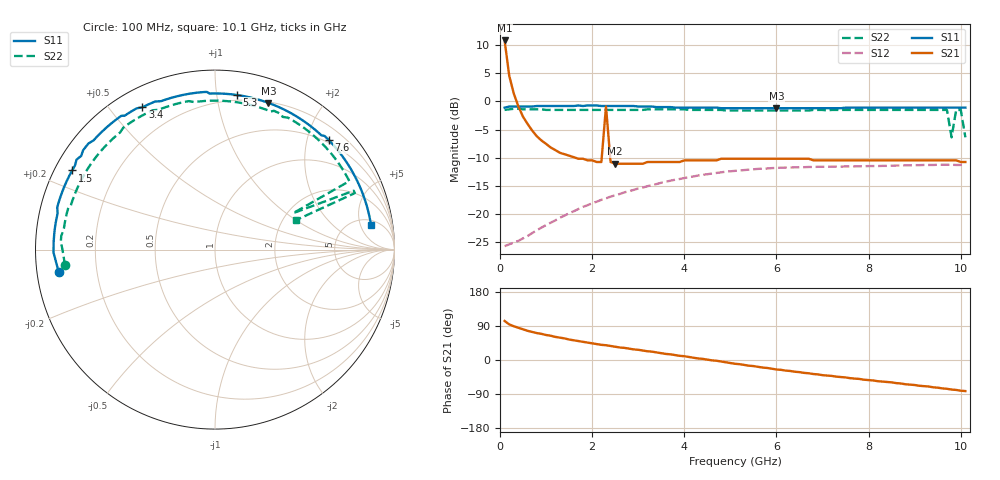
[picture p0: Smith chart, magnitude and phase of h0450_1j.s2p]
!HBFP-0450
!S and NOISE PARAMETERS at Vce=1V  Ic=100mA.  LAST UPDATED  09-04-98
# GHZ S MA R  50
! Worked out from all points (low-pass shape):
!   101 points, 100 MHz to 10.1 GHz, reference 50 ohm
!   highest |S21| = 10.81 dB at 100 MHz (marker M1); lowest = -11.1 dB at 2.5 GHz (marker M2)
!   |S21| within 3 dB of the highest: start of sweep to 148 MHz
!   lowest |S11| = -1.2 dB at 6 GHz (marker M3), VSWR 14.38, Z = 10.5 + j70.4 ohm
!   |S11| at or under -10 dB: nowhere
!   |S22| runs from -6.4 to -1.3 dB; largest |S21 - S12| = 3.5
!   S11 on the Smith chart (normalised r, x): 100 MHz: 0.06, -0.07; 1.5 GHz: 0.05, +0.26; 3.4 GHz: 0.08, +0.61; 5.3 GHz: 0.16, +1.14; 7.6 GHz: 0.44, +2.40; 10.1 GHz: 6.25, +7.63
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0.1  0.88 -172.0  3.47 103.0  0.052 12.0  0.84 -174.0
0.2  0.9 -179.0  1.69 94.0  0.054 13.0  0.85 -180.0
0.4  0.9 174.0  0.9 85.0  0.058 19.0  0.86 175.0
0.8  0.91 165.0  0.49 71.0  0.072 27.0  0.85 166.0
1.5  0.91 151.0  0.33 54.0  0.102 32.0  0.84 154.0
1.8  0.91 145.0  0.31 48.0  0.116 31.0  0.84 149.0
2.2  0.91 138.0  0.29 40.0  0.134 29.0  0.84 142.0
2.3  0.91 136.0  0.9 39.0  0.138 28.0  0.84 141.0
2.4  0.91 134.0  0.29 37.0  0.143 27.0  0.84 139.0
2.5  0.91 132.0  0.28 35.0  0.147 26.0  0.84 138.0
3.4  0.89 117.0  0.29 20.0  0.185 16.0  0.85 124.0
3.5  0.89 115.0  0.29 18.0  0.19 14.0  0.85 122.0
5.1  0.87 86.0  0.31 -10.0  0.242 -10.0  0.83 94.0
5.3  0.87 82.0  0.31 -13.0  0.246 -13.0  0.83 91.0
6  0.87 70.0  0.31 -25.0  0.257 -24.0  0.83 79.0
6.8  0.87 56.0  0.3 -37.0  0.262 -36.0  0.84 67.0
7.6  0.88 44.0  0.3 -48.0  0.265 -47.0  0.84 56.0
8.5  0.88 31.0  0.3 -59.0  0.269 -58.0  0.84 44.0
9.7  0.88 15.0  0.3 -76.0  0.274 -75.0  0.84 27.0
9.8  0.88 13.0  0.3 -78.0  0.274 -76.0  0.48 25.0
10  0.88 10.0  0.29 -81.0  0.273 -79.0  0.84 22.0
10.1  0.88 9.0  0.29 -82.0  0.272 -81.0  0.48 20.0
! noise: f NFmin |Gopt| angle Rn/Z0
1.8  2.89  0.8  -151  0.27
2  2.89  0.84  -146  0.36
2.5  2.87  0.81  -138  0.51
3.5  2.82  0.77  -121  0.77
4  2.78  0.75  -113  0.89
5  2.76  0.76  -94  1.19
5.5  2.72  0.74  -85  1.37
7  2.65  0.79  -57  2.04
8  2.59  0.77  -43  2.07
10  2.53  0.83  -14  2.86
